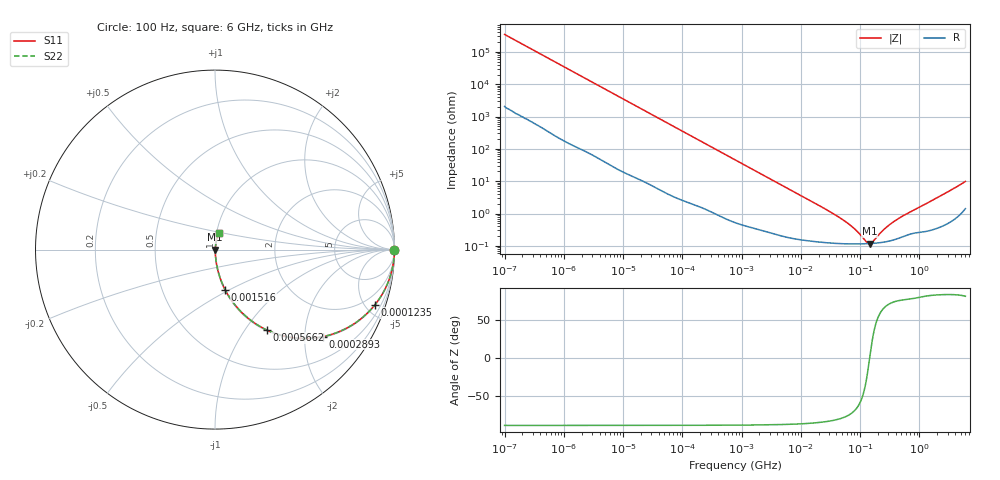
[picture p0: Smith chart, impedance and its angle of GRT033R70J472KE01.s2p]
!Murata Part Number: GRT033R70J472KE01
!These Parameters are Measured in Series Mode Connection
!Data Generated on Jun 19, 2026
!  o--ll--o
!Port1  Port2
!  o------o
!Operation Temp=25[degC], DC Bias Voltage=0[V]
!Freq. Start=100[Hz] Stop=6[GHz] 401[Steps]
# Hz S RI R 50
!Freq.(Hz) S11(Real) S11(Imag) S21(Real) S21(Imag) S12(Real) S12(Imag) S22(Real) S22(Imag)
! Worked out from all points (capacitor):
!   401 points, 100 Hz to 6 GHz, reference 50 ohm
!   read as one part in series: C = 4.59 nF near 109 Hz
!   lowest |Z| = 118 mohm at 145.9 MHz (marker M1)
!   series resonance near 145.3 MHz, so ESL is about 260 pH
!   S11 on the Smith chart (normalised r, x): 100 Hz: open; 123.5 kHz: 1.04, -5.74; 289.3 kHz: 1.02, -2.47; 566.2 kHz: 1.01, -1.26; 1.516 MHz: 1.01, -0.47; 6 GHz: 1.03, +0.20
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100  1 -0.000289  1.8e-06 0.000289  1.8e-06 0.000289  1 -0.000289
2008  0.9999 -0.00574  6.41e-05 0.00574  6.41e-05 0.00574  0.9999 -0.00574
12592  0.9985 -0.0357  0.00148 0.0357  0.00148 0.0357  0.9985 -0.0357
40335  0.9864 -0.1125  0.0136 0.1125  0.0136 0.1125  0.9864 -0.1125
123542  0.89 -0.309  0.11 0.309  0.11 0.309  0.89 -0.309
184852  0.7852 -0.4063  0.2148 0.4063  0.2148 0.4063  0.7852 -0.4063
289253  0.6022 -0.4847  0.3978 0.4847  0.3978 0.4847  0.6022 -0.4847
395726  0.4496 -0.4925  0.5504 0.4925  0.5504 0.4925  0.4496 -0.4925
566185  0.2876 -0.4474  0.7124 0.4474  0.7124 0.4474  0.2876 -0.4474
774597  0.1791 -0.3779  0.8209 0.3779  0.8209 0.3779  0.1791 -0.3779
1516199  0.0563 -0.2231  0.9437 0.2231  0.9437 0.2231  0.0563 -0.2231
4060267  0.01 -0.0882  0.99 0.0882  0.99 0.0882  0.01 -0.0882
1.555665e7  0.00193 -0.0232  0.9981 0.0232  0.9981 0.0232  0.00193 -0.0232
5.699437e7  0.00119 -0.00548  0.9988 0.00548  0.9988 0.00548  0.00119 -0.00548
8.527865e7  0.00116 -0.00284  0.9988 0.00284  0.9988 0.00284  0.00116 -0.00284
1.275994e8  0.00117 -0.000663  0.9988 0.000663  0.9988 0.000663  0.00117 -0.000663
1.459435e8  0.00118 2.12e-05  0.9988 -2.12e-05  0.9988 -2.12e-05  0.00118 2.12e-05
1.669249e8  0.0012 0.000705  0.9988 -0.000705  0.9988 -0.000705  0.0012 0.000705
2.388273e8  0.00129 0.00262  0.9987 -0.00262  0.9987 -0.00262  0.00129 0.00262
3.124326e8  0.00143 0.00424  0.9986 -0.00424  0.9986 -0.00424  0.00143 0.00424
5.59173e8  0.00208 0.0087  0.9979 -0.0087  0.9979 -0.0087  0.00208 0.0087
6e9  0.023 0.094  0.977 -0.094  0.977 -0.094  0.023 0.094
